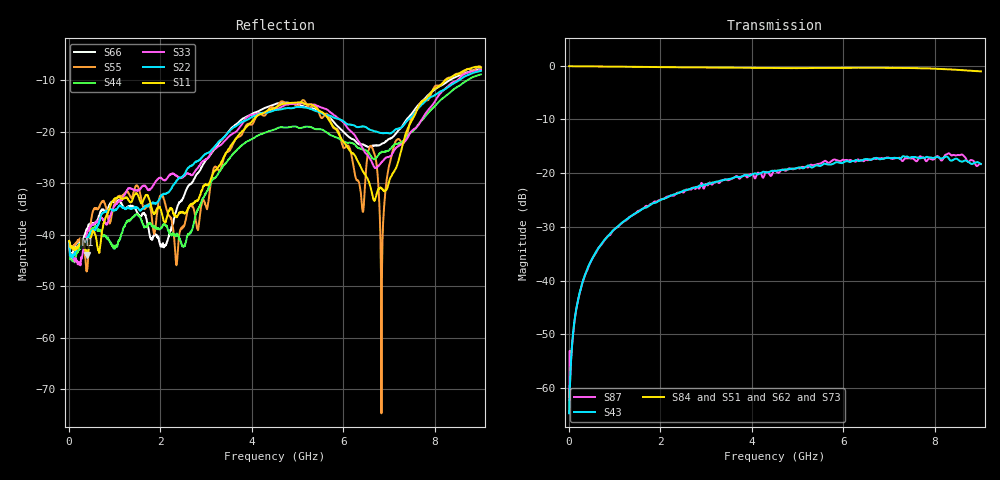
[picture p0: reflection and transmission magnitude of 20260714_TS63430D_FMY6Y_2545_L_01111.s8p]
# GHz S DB R 50
! CMT, SN0916, 25263762, 26.7.0
! Date: 15.07.2026 14:59:59
! Data: Format
! Freq S1.1:dB/Ang S1.2:dB/Ang S1.3:dB/Ang S1.4:dB/Ang S1.5:dB/Ang S1.6:dB/Ang S1.7:dB/Ang S1.8:dB/Ang
!  S2.1:dB/Ang S2.2:dB/Ang S2.3:dB/Ang S2.4:dB/Ang S2.5:dB/Ang S2.6:dB/Ang S2.7:dB/Ang S2.8:dB/Ang
!  S3.1:dB/Ang S3.2:dB/Ang S3.3:dB/Ang S3.4:dB/Ang S3.5:dB/Ang S3.6:dB/Ang S3.7:dB/Ang S3.8:dB/Ang
!  S4.1:dB/Ang S4.2:dB/Ang S4.3:dB/Ang S4.4:dB/Ang S4.5:dB/Ang S4.6:dB/Ang S4.7:dB/Ang S4.8:dB/Ang
!  S5.1:dB/Ang S5.2:dB/Ang S5.3:dB/Ang S5.4:dB/Ang S5.5:dB/Ang S5.6:dB/Ang S5.7:dB/Ang S5.8:dB/Ang
!  S6.1:dB/Ang S6.2:dB/Ang S6.3:dB/Ang S6.4:dB/Ang S6.5:dB/Ang S6.6:dB/Ang S6.7:dB/Ang S6.8:dB/Ang
!  S7.1:dB/Ang S7.2:dB/Ang S7.3:dB/Ang S7.4:dB/Ang S7.5:dB/Ang S7.6:dB/Ang S7.7:dB/Ang S7.8:dB/Ang
!  S8.1:dB/Ang S8.2:dB/Ang S8.3:dB/Ang S8.4:dB/Ang S8.5:dB/Ang S8.6:dB/Ang S8.7:dB/Ang S8.8:dB/Ang
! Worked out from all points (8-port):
!   2001 points, 10 MHz to 9 GHz, reference 50 ohm
!   strongest paths, dB at 10 MHz, 2.257 GHz, 4.505 GHz, 6.753 GHz, 9 GHz:
!     S84: -0.1, -0.3, -0.4, -0.4, -1.0
!     S51: -0.1, -0.2, -0.5, -0.4, -1.3
!     S62: -0.1, -0.3, -0.5, -0.4, -1.2
!     S73: -0.1, -0.3, -0.6, -0.4, -1.2
!     S43: -64.7, -24.1, -19.6, -17.3, -18.3
!     S87: -61.5, -24.2, -19.5, -17.2, -18.3
!   lowest |S11| = -43.9 dB at 410.1 MHz (marker M1), VSWR 1.01, Z = 50.3 - j0.579 ohm
!   |S11| at or under -10 dB: start of sweep to 8.236 GHz
